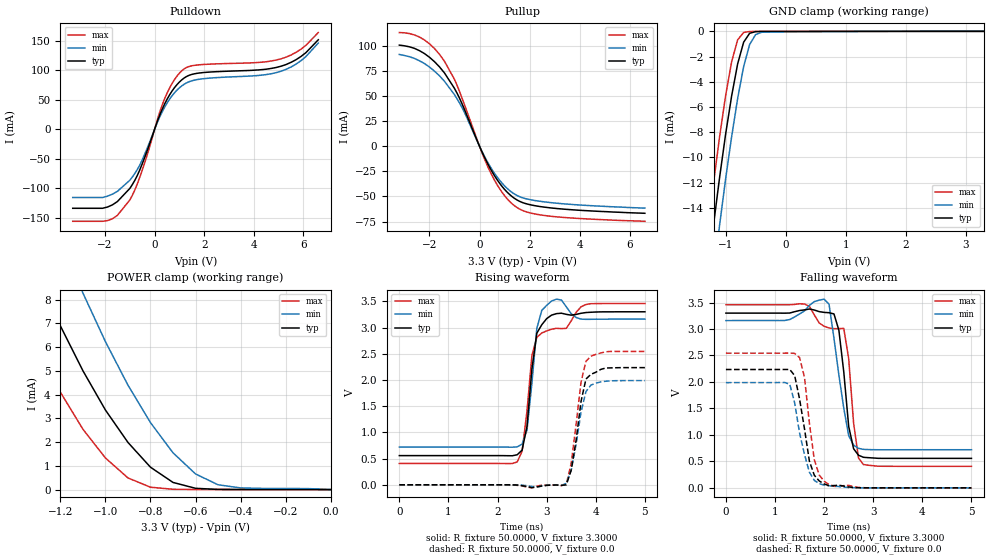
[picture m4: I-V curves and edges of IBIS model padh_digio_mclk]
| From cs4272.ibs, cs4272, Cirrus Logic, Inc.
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|   Model mclk
[Model]  padh_digio_mclk
Model_type I/O
Polarity   Non-Inverting
Enable   Active-High
Vinl =   0.8000V
Vinh =   2.0000V
C_comp   5.0000pF   5.0000pF   5.0000pF
[Temperature Range]   25.0000   85.0000   -40.0000
[Voltage Range]   3.3000V   3.0000V   3.6000V
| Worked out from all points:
|   slope of the pulldown table from 0 to 0.495 V, typ, clamps not added: 9.86 ohm
|   slope of the pullup table from 0 to 0.495 V, typ, clamps not added: 19.8 ohm
|   GND clamp passes 1 mA (typ) near -0.71 V on its own axis
|   POWER clamp passes 1 mA (typ) near -0.81 V on its own axis
|   rising waveform, R_fixture 50.0000, V_fixture 3.3000: 20-80 % time 182ps typ, 152ps min, 294ps max; typ from 0.557 V to 3.3 V
|   rising waveform, R_fixture 50.0000, V_fixture 0.0: 20-80 % time 217ps typ, 227ps min, 206ps max; typ from 0 V to 2.23 V
|   falling waveform, R_fixture 50.0000, V_fixture 3.3000: 20-80 % time 184ps typ, 235ps min, 203ps max; typ from 3.3 V to 0.557 V
|   falling waveform, R_fixture 50.0000, V_fixture 0.0: 20-80 % time 246ps typ, 267ps min, 201ps max; typ from 2.23 V to 0 V
[Pulldown]
|Voltage   I(typ)   I(min)   I(max)
-3.3V     -133.6mA   -115.4mA   -155.6mA
-2.1V     -133.6mA   -115.4mA   -155.6mA
-1.7V     -127.8mA   -109.7mA   -151.4mA
-1V       -100.1mA   -86.22mA   -119.6mA
-500mV    -58.64mA   -51.91mA   -69.38mA
400mV     42.38mA    37.02mA    51.17mA
800mV     70.37mA    61.68mA    84.01mA
1.2V      87.06mA    76.45mA    102.6mA
1.8V      95.27mA    84.7mA     109.2mA
5.1V      106.8mA    98.33mA    119.3mA
5.9V      123.2mA    116.1mA    135.5mA
6.6V      151.5mA    146mA      163.7mA
[Pullup]
|Voltage   I(typ)   I(min)   I(max)
-3.2V     100.5mA    91.24mA    113mA
-2.2V     92.16mA    82.22mA    105.7mA
-1.4V     72.91mA    64.63mA    84.57mA
-1V       57.55mA    51.28mA    66.47mA
-700mV    42.4mA     38.53mA    48.02mA
100mV     -5.681mA   -5.222mA   -6.579mA
400mV     -20.83mA   -19.15mA   -24.02mA
900mV     -40mA      -36.76mA   -45.84mA
1.4V      -51.95mA   -47.65mA   -59.28mA
1.9V      -57.47mA   -52.52mA   -65.5mA
2.7V      -60.95mA   -55.69mA   -69.24mA
6.6V      -66.7mA    -61.6mA    -74.68mA
[GND_clamp]
|Voltage   I(typ)   I(min)   I(max)
-3.3V     -106.5mA   -109mA     -107mA
-1.3V     -19.2mA    -23.21mA   -15.94mA
-1.2V     -15.29mA   -19.2mA    -11.99mA
-1.1V     -11.57mA   -15.35mA   -8.336mA
-1V       -8.148mA   -11.7mA    -5.089mA
-900mV    -5.124mA   -8.356mA   -2.406mA
-800mV    -2.578mA   -5.329mA   -667.5uA
-700mV    -856.5uA   -2.792mA   -82.16uA
-600mV    -148.4uA   -1.042mA   -6.83uA
-500mV    -14.48uA   -249.7uA   -2.318uA
-400mV    -2.151uA   -66.74uA   -1.738uA
3.3V      3.357uA    49.76uA    4.351uA
[POWER_clamp]
|Voltage   I(typ)   I(min)   I(max)
-3.3V     67.56mA    73.96mA    64.01mA
-1.4V     11.23mA    15.43mA    7.976mA
-1.3V     8.974mA    12.9mA     5.923mA
-1.2V     6.887mA    10.51mA    4.097mA
-1.1V     5.001mA    8.273mA    2.54mA
-1V       3.348mA    6.226mA    1.33mA
-900mV    1.985mA    4.396mA    491.5uA
-800mV    942.6uA    2.82mA     100.1uA
-700mV    302.3uA    1.55mA     13.84uA
-600mV    55.15uA    660.5uA    4.906uA
-400mV    3.685uA    71.39uA    4.356uA
0V        0A         0A         0A
[Ramp]
| variable   typ   min   max
dV/dt_r  1.3410/0.2371n   1.0956/0.2934n   1.6002/0.1834n
dV/dt_f  1.6459/0.1595n   1.4015/0.2008n   1.8901/0.1126n
R_load = 50.0000
[Rising Waveform]
R_fixture= 50.0000
V_fixture= 3.3000
V_fixture_min= 3.6000
V_fixture_max= 3.0000
|time   V(typ)   V(min)   V(max)
0s        556.7mV    720.1mV    406.8mV
2.4ns     572.8mV    723.4mV    435.5mV
2.5ns     661.5mV    776.1mV    639.4mV
2.6ns     1.117V     1.044V     1.409V
2.7ns     2.211V     1.94V      2.47V
2.8ns     2.892V     2.985V     2.812V
3ns       3.17V      3.424V     2.936V
3.4ns     3.251V     3.396V     2.985V
3.8ns     3.286V     3.156V     3.438V
5ns       3.3V       3.16V      3.458V
[Rising Waveform]
R_fixture= 50.0000
V_fixture= 0.0
|time   V(typ)   V(min)   V(max)
0s        0V         252.7uV    0V
2.7ns     -54.02mV   -32.94mV   -58.3mV
3.4ns     120uV      26.66mV    11.98mV
3.5ns     280.9mV    278mV      410.6mV
3.6ns     850.9mV    770.1mV    1.154V
3.7ns     1.591V     1.389V     1.959V
3.8ns     2.017V     1.778V     2.354V
3.9ns     2.106V     1.901V     2.453V
4.2ns     2.227V     1.975V     2.537V
5ns       2.235V     1.988V     2.544V
[Falling Waveform]
R_fixture= 50.0000
V_fixture= 3.3000
V_fixture_min= 3.6000
V_fixture_max= 3.0000
|time   V(typ)   V(min)   V(max)
0s        3.3V       3.159V     3.458V
1.6ns     3.361V     3.342V     3.473V
2ns       3.313V     3.564V     3.051V
2.1ns     3.307V     3.468V     3.019V
2.2ns     3.285V     2.828V     3.006V
2.4ns     2.189V     1.504V     3.011V
2.5ns     1.16V      986mV      2.439V
2.6ns     739mV      806.9mV    1.222V
2.8ns     577.3mV    727mV      440.6mV
5ns       556.8mV    719.8mV    406.8mV
[Falling Waveform]
R_fixture= 50.0000
V_fixture= 0.0
|time   V(typ)   V(min)   V(max)
0s        2.235V     1.987V     2.544V
1.3ns     2.236V     1.956V     2.545V
1.4ns     2.12V      1.606V     2.54V
1.5ns     1.677V     1.036V     2.46V
1.6ns     1.115V     632.2mV    2.091V
1.7ns     503.7mV    296.6mV    1.22V
1.8ns     238.5mV    141.2mV    530.8mV
1.9ns     130.2mV    79.8mV     243.9mV
2.1ns     40.3mV     38.72mV    61.25mV
5ns       -10.46uV   0V         1.837uV
